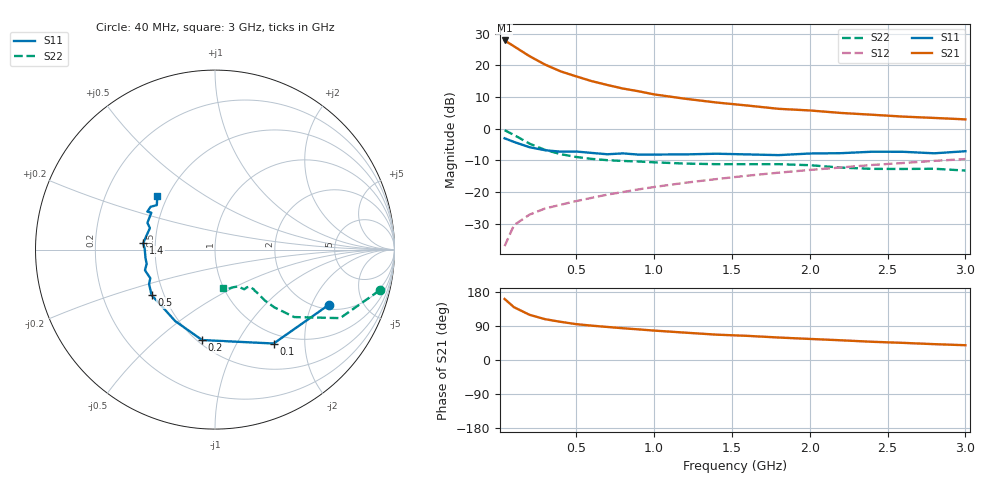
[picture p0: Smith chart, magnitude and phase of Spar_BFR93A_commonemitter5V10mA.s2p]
! Filename:  BFR93AB.S2P  Version:  2.0
! NXP part #: BFR93A  Date: May 1990
! Bias condition: Vce=5V, Ic=10mA
#  MHz  S  MA  R  50
! Freq  S11  S21  S12  S22  !GUM [dB]
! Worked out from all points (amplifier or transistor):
!   21 points, 40 MHz to 3 GHz, reference 50 ohm
!   highest |S21| = 27.8 dB at 40 MHz (marker M1)
!   |S21| within 3 dB of that: start of sweep to 137.4 MHz
!   unconditionally stable (mu >= 1): 910.9 MHz to 2.916 GHz
!   at 300 MHz: K = 0.66, MSG = 22.7 dB, |S12| = -25.2 dB
!   at 1 GHz: K = 1.02, MAG = 13.7 dB, |S12| = -18.4 dB
!   at 3 GHz: K = 0.99, MSG = 6.3 dB, |S12| = -9.6 dB
!   S11 on the Smith chart (normalised r, x): 40 MHz: 2.19, -2.68; 100 MHz: 0.85, -1.44; 200 MHz: 0.53, -0.72; 500 MHz: 0.43, -0.27; 1.4 GHz: 0.43, +0.04; 3 GHz: 0.44, +0.33
40  0.704 -26.0  24.58 161.0  0.014 77.0  0.945 -13.9
100  0.617 -58.0  19.89 139.4  0.03 64.2  0.795 -28.7
200  0.509 -98.1  13.9 119.3  0.044 57.3  0.58 -40.4
300  0.456 -119.1  10.22 107.7  0.055 56.0  0.462 -44.2
400  0.433 -133.1  7.994 100.7  0.063 57.6  0.396 -45.6
500  0.435 -144.4  6.667 94.6  0.072 58.9  0.357 -45.6
600  0.414 -152.5  5.609 90.6  0.081 61.1  0.333 -45.7
700  0.394 -156.2  4.879 87.2  0.091 62.8  0.318 -46.0
800  0.407 -163.5  4.286 83.8  0.1 64.0  0.309 -45.7
900  0.389 -168.2  3.888 80.8  0.11 65.1  0.303 -46.0
1000  0.39 -173.0  3.469 77.6  0.12 66.0  0.294 -46.2
1200  0.392 179.2  2.959 72.2  0.14 66.8  0.281 -47.2
1400  0.402 175.0  2.583 66.9  0.16 67.1  0.275 -50.0
1600  0.392 170.1  2.312 63.7  0.181 67.5  0.275 -51.7
1800  0.382 161.7  2.053 59.3  0.202 67.0  0.275 -53.5
2000  0.405 158.4  1.935 55.6  0.223 66.8  0.265 -54.8
2200  0.41 149.9  1.767 52.0  0.244 66.5  0.243 -57.7
2400  0.432 150.7  1.656 48.1  0.267 65.4  0.232 -64.9
2600  0.431 146.4  1.547 45.2  0.287 64.1  0.231 -71.0
2800  0.408 142.6  1.474 41.8  0.31 63.5  0.233 -74.8
3000  0.44 136.9  1.399 39.0  0.331 61.8  0.218 -77.7
